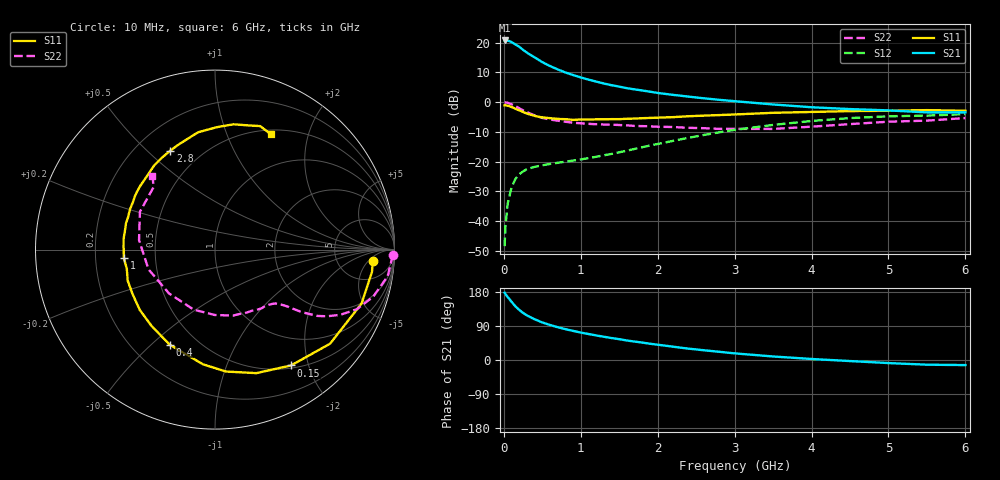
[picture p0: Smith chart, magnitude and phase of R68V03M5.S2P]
! SIEMENS Small Signal Semiconductors
! BFR193
! Si NPN RF Bipolar Junction Transistor in SOT23
! VCE = 8 V  IC = 3.5 mA
! Common Emitter S-Parameters:  May  1996
# GHz  S  MA  R  50
!  f  S11  S21  S12  S22
! GHz  MAG  ANG  MAG  ANG  MAG  ANG  MAG  ANG
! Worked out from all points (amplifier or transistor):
!   36 points, 10 MHz to 6 GHz, reference 50 ohm
!   highest |S21| = 20.7 dB at 10 MHz (marker M1)
!   |S21| within 3 dB of that: start of sweep to 242.2 MHz
!   unconditionally stable (mu >= 1): 1.028 GHz to 2.066 GHz
!   at 250 MHz: K = 0.33, MSG = 20.4 dB, |S12| = -23.3 dB
!   at 1.4 GHz: K = 1.08, MAG = 9.8 dB, |S12| = -17.4 dB
!   at 6 GHz: K = 0.97, MSG = 0.3 dB, |S12| = -4.0 dB
!   S11 on the Smith chart (normalised r, x): 10 MHz: 12, -7; 150 MHz: 0.54, -1.72; 400 MHz: 0.35, -0.57; 1 GHz: 0.33, -0.04; 2.8 GHz: 0.34, +0.59; 6 GHz: 0.55, +1.45
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0.01  0.8822 -4.1  10.84 177.5  0.0038 86.7  0.9932 -1.8
0.02  0.8834 -8.1  10.78 174.3  0.0079 84.5  0.9852 -3.5
0.05  0.8702 -20.2  10.82 166.3  0.0197 78.3  0.9734 -8.8
0.1  0.8281 -39.3  10.19 153.7  0.0368 70.3  0.9196 -16.6
0.15  0.7721 -56.7  9.322 141.6  0.0511 61.6  0.8571 -22.8
0.2  0.7258 -71.5  8.495 132.2  0.0612 55.8  0.7871 -27.5
0.25  0.6821 -84.9  7.532 124.3  0.0684 50.8  0.7257 -30.8
0.3  0.6425 -96.0  6.775 117.7  0.0748 47.8  0.6783 -33.0
0.4  0.5867 -115.5  5.629 107.4  0.0817 43.7  0.5979 -35.7
0.5  0.5529 -129.8  4.689 99.1  0.0867 42.6  0.5418 -37.3
0.6  0.5372 -141.3  4.029 92.4  0.0914 42.1  0.5094 -38.3
0.8  0.5163 -160.4  3.146 81.4  0.0997 43.9  0.4672 -40.6
1  0.5098 -174.6  2.595 72.5  0.1087 48.2  0.44 -43.4
1.1  0.5093 178.8  2.386 68.6  0.1146 50.1  0.4313 -45.3
1.3  0.5126 168.2  2.052 61.4  0.1277 53.4  0.4196 -49.1
1.6  0.5244 154.6  1.711 51.5  0.1527 57.6  0.4064 -56.3
2.2  0.5585 132.6  1.322 35.1  0.2232 59.7  0.3812 -74.5
2.8  0.605 114.2  1.092 21.7  0.3107 54.9  0.3545 -99.5
3.5  0.6605 98.2  0.912 9.3  0.4135 44.2  0.3538 -136.4
4.5  0.7056 81.6  0.763 -2.8  0.5385 26.2  0.4265 172.9
5.5  0.7326 69.9  0.671 -12.4  0.5924 8.0  0.4882 134.5
6  0.714 64.0  0.671 -13.4  0.6275 2.9  0.5397 130.2
